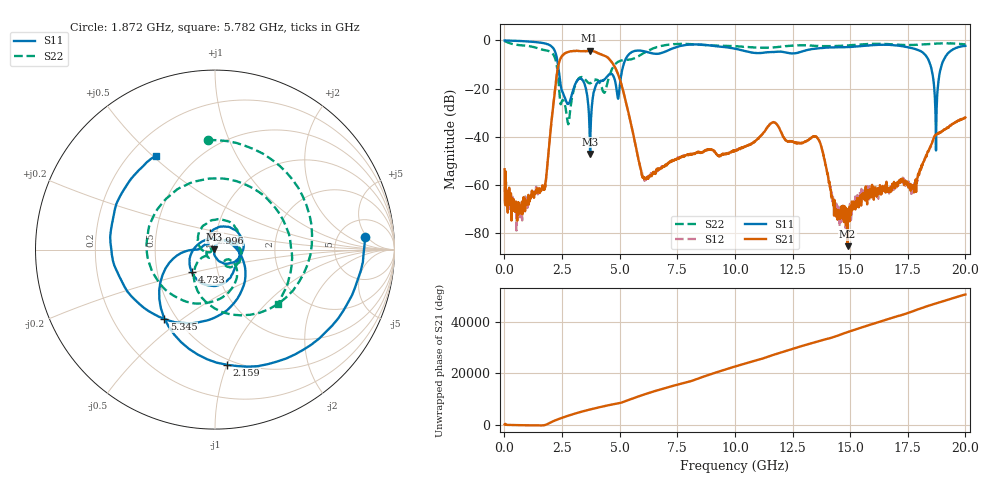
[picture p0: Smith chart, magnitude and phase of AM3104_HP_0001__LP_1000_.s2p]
!Created with skrf (http://scikit-rf.org).
# Hz S RI R 50.0
!freq ReS11 ImS11 ReS21 ImS21 ReS12 ImS12 ReS22 ImS22
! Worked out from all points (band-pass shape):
!   1601 points, 10 MHz to 20 GHz, reference 50 ohm
!   highest |S21| = -4.25 dB at 3.696 GHz (marker M1); lowest = -85.5 dB at 14.89 GHz (marker M2)
!   |S21| within 3 dB of the highest: 2.449 GHz to 4.503 GHz (2.053 GHz wide, 59.1 % of centre)
!   lowest |S11| = -47.1 dB at 3.721 GHz (marker M3), VSWR 1.01, Z = 49.6 + j0.253 ohm
!   |S11| at or under -10 dB: 2.325 GHz to 5.171 GHz (2.846 GHz wide, 75.9 % of centre); 18.48 GHz to 18.98 GHz (501.3 MHz wide, 2.68 % of centre)
!   |S22| runs from -34.8 to -0.2 dB; largest |S21 - S12| = 0.0046
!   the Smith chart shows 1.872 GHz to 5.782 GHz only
!   S11 on the Smith chart (normalised r, x): 1.872 GHz: 9, +4; 2.159 GHz: 0.46, -1.00; 2.996 GHz: 0.93, +0.18; 4.733 GHz: 0.75, -0.20; 5.345 GHz: 0.43, -0.43; 5.782 GHz: 0.30, +0.51
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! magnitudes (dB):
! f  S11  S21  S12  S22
! 10 MHz  0.0  -53.5  -61.0  -0.2
! 647.2 MHz  -0.2  -69.3  -70.5  -1.9
! 1.872 GHz  -1.5  -51.2  -51.1  -4.3
! 2.159 GHz  -3.8  -23.3  -23.2  -6.4
! 2.734 GHz  -26.4  -4.9  -4.9  -33.3
! 2.996 GHz  -20.2  -4.4  -4.3  -21.0
! 3.346 GHz  -15.9  -4.5  -4.5  -15.2
! 3.696 GHz  -37.2  -4.3  -4.3  -17.8
! 3.721 GHz  -47.1  -4.3  -4.2  -17.8
! 4.008 GHz  -17.9  -5.0  -5.0  -16.3
! 4.733 GHz  -14.9  -10.1  -10.1  -10.8
! 5.345 GHz  -6.4  -28.5  -28.5  -8.0
! 5.782 GHz  -4.2  -48.0  -48.0  -6.7
! 6.682 GHz  -5.5  -53.6  -54.0  -2.6
! 10.01 GHz  -3.4  -45.9  -45.7  -2.4
! 13.34 GHz  -3.5  -40.2  -40.2  -2.2
! 14.89 GHz  -2.8  -85.5  -72.7  -2.0
! 16.68 GHz  -1.8  -61.6  -60.4  -1.5
! 18.25 GHz  -5.9  -48.8  -49.1  -1.6
! 18.73 GHz  -45.7  -39.2  -39.2  -1.3
! 19.09 GHz  -7.5  -37.1  -36.9  -1.2
! 20 GHz  -2.3  -32.0  -32.1  -1.6
